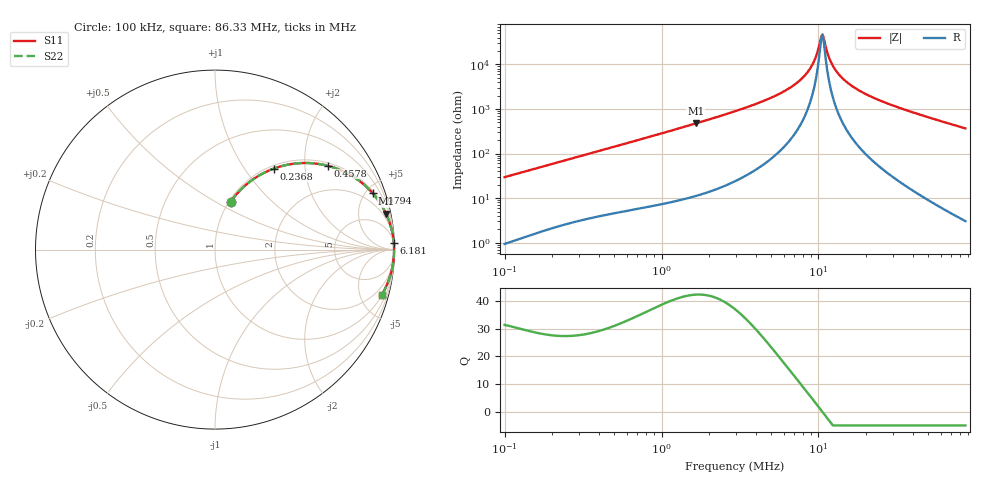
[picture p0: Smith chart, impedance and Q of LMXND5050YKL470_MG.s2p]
! LMXND5050YKL470_MG  S-PARAMETER MODEL  ( General Type )
! Model Generated by TAIYO YUDEN Corporation (https://www.yuden.co.jp/en/)
! Version 1.0
! TAIYO YUDEN Control No. 191023NI43SB-FBB
! Copyright(c) 2019 TAIYO YUDEN CO.,LTD. All Rights Reserved.
! Product Description (link to TY-COMPAS)
! https://ds.yuden.co.jp/TYCOMPAS/or/detail?pn=LMXND5050YKL470MMG&u=M
! Products Name : Inductors
! Characteristics :
!  Inductance : 47 uH , SRF(min) : 6.0 MHz , DC Resistance(max) : 0.403 Ohm
!  Rated Current : Saturation :1100 mA , Temp Rise : 900 mA (40 degC)
!  Case Size : 4.9 x 4.9 / 0.193 x 0.193 [mm/inch] , Thickness : 4 / 0.157 [mm/inch]
!  (Conditions: Temperature = 25 degC , DC Bias Current/Voltage = 0A / 0V)
! External Node Assignments :
!  1  o---GGG---o  2
! GND o---------o GND
! Frequency Range : 0.1MHz  -  86.325287MHz  [ 402 STEP ]
# MHz S RI R 50
! Freq[MHz].  S11 Real  S11 Imag  S21 Real  S21 Imag  S12 Real  S12 Imag  S22 Real  S22 Imag
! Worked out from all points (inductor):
!   401 points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, 100 kHz to 86.33 MHz, reference 50 ohm
!   read as one part in series: L = 46.9 uH near 103.4 kHz
!   highest Q = 42.4 at 1.654 MHz (marker M1), where L = 45.7 uH
!   self-resonance near 10.44 MHz
!   S11 on the Smith chart (normalised r, x): 100 kHz: 1.02, +0.59; 236.8 kHz: 1.05, +1.37; 457.8 kHz: 1.09, +2.61; 979.4 kHz: 1.14, +5.56; 6.181 MHz: 4, +52; 86.33 MHz: 1.06, -7.34
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0.1  0.0877 0.2674  0.9123 -0.2674  0.9123 -0.2674  0.0877 0.2674
0.236787  0.3269 0.4512  0.6731 -0.4512  0.6731 -0.4512  0.3269 0.4512
0.310315  0.4463 0.4795  0.5537 -0.4795  0.5537 -0.4795  0.4463 0.4795
0.457753  0.6268 0.4674  0.3732 -0.4674  0.3732 -0.4674  0.6268 0.4674
0.962956  0.8755 0.3173  0.1245 -0.3173  0.1245 -0.3173  0.8755 0.3173
0.97937  0.8791 0.3133  0.1209 -0.3133  0.1209 -0.3133  0.8791 0.3133
1.653854  0.9532 0.1998  0.0468 -0.1998  0.0468 -0.1998  0.9532 0.1998
2.938117  0.9846 0.1104  0.0154 -0.1104  0.0154 -0.1104  0.9846 0.1104
4.559508  0.9935 0.0634  0.0065 -0.0634  0.0065 -0.0634  0.9935 0.0634
6.180793  0.9963 0.038  0.00371 -0.038  0.00371 -0.038  0.9963 0.038
7.830852  0.9974 0.0206  0.0026 -0.0206  0.0026 -0.0206  0.9974 0.0206
9.117424  0.9978 0.0101  0.00224 -0.0101  0.00224 -0.0101  0.9978 0.0101
9.591647  0.9978 0.00661  0.00217 -0.00661  0.00217 -0.00661  0.9978 0.00661
10.26253  0.9979 0.00204  0.00212 -0.00204  0.00212 -0.00204  0.9979 0.00204
10.61537  0.9979 -0.000246  0.00211 0.000246  0.00211 0.000246  0.9979 -0.000246
10.79632  0.9979 -0.00139  0.00211 0.00139  0.00211 0.00139  0.9979 -0.00139
11.55146  0.9979 -0.00596  0.00214 0.00596  0.00214 0.00596  0.9979 -0.00596
12.15229  0.9978 -0.0094  0.00218 0.0094  0.00218 0.0094  0.9978 -0.0094
14.14885  0.9975 -0.0199  0.00248 0.0199  0.00248 0.0199  0.9975 -0.0199
18.54243  0.9963 -0.0399  0.00366 0.0399  0.00366 0.0399  0.9963 -0.0399
28.29276  0.9919 -0.0772  0.00807 0.0772  0.00807 0.0772  0.9919 -0.0772
86.32529  0.9291 -0.2526  0.0709 0.2526  0.0709 0.2526  0.9291 -0.2526
